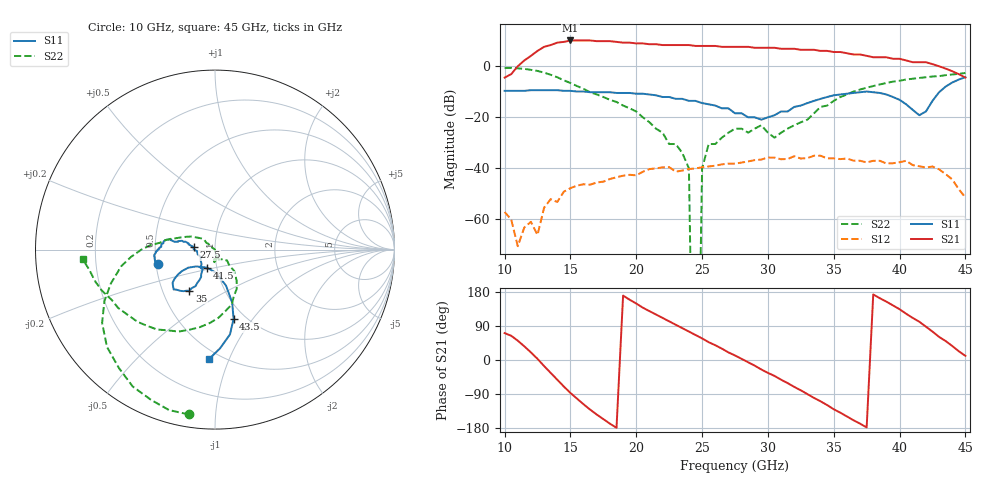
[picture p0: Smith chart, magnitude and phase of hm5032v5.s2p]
!  HMMC-5032
!  S-PARAMETERS at Vdd = 4.5V, Idd = 250mA  LAST UPDATED 03-10-98
#  GHZ  S  MA  R 50
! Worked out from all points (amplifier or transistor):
!   71 points, 10 GHz to 45 GHz, reference 50 ohm
!   highest |S21| = 10.1 dB at 15 GHz (marker M1)
!   |S21| within 3 dB of that: 12.84 GHz to 30.67 GHz (17.83 GHz wide, 81.9 % of centre)
!   unconditionally stable (mu >= 1): start of sweep to end of sweep
!   at 15.5 GHz: K = 25.30, MAG = 11.4 dB, |S12| = -46.7 dB
!   at 27.5 GHz: K = 16.51, MAG = 7.7 dB, |S12| = -38.1 dB
!   at 45 GHz: K = 87.25, MAG = 1.0 dB, |S12| = -51.4 dB
!   S11 on the Smith chart (normalised r, x): 10 GHz: 0.51, -0.09; 27.5 GHz: 0.79, +0.02; 35 GHz: 0.68, -0.34; 41.5 GHz: 0.90, -0.18; 43.5 GHz: 0.88, -0.81; 45 GHz: 0.44, -0.85
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10  0.33 -166.0  0.6 71.0  0.0014 -173.0  0.93 -99.0
11.5  0.33 -167.0  1.3 36.0  0.0007 -143.0  0.89 -121.0
13  0.34 -172.0  2.4 -16.0  0.0017 -134.0  0.75 -147.0
14  0.34 -175.0  2.9 -52.0  0.0022 -168.0  0.61 -162.0
15  0.33 -178.0  3.2 -87.0  0.0041 171.0  0.47 -175.0
16  0.32 -180.0  3.2 -117.0  0.0049 147.0  0.36 176.0
18.5  0.3 177.0  3 -179.0  0.0067 118.0  0.2 160.0
20.5  0.29 171.0  2.8 138.0  0.0086 95.0  0.1 141.0
22  0.25 167.0  2.6 111.0  0.0105 63.0  0.05 139.0
24  0.21 168.0  2.6 75.0  0.0097 45.0  0.01 146.0
24.5  0.21 167.0  2.5 66.0  0.01 41.0  0 -112.0
25  0.19 165.0  2.5 57.0  0.0105 36.0  0.01 -88.0
25.5  0.18 166.0  2.5 47.0  0.0109 30.0  0.03 -72.0
27.5  0.12 173.0  2.4 12.0  0.0124 7.0  0.06 -83.0
30.5  0.11 -133.0  2.3 -42.0  0.0163 -39.0  0.04 -88.0
33.5  0.21 -118.0  2.1 -100.0  0.0177 -90.0  0.12 -48.0
35  0.27 -122.0  1.9 -130.0  0.0157 -115.0  0.21 -55.0
37  0.31 -134.0  1.7 -168.0  0.0141 -152.0  0.35 -81.0
39.5  0.25 -146.0  1.4 144.0  0.0126 160.0  0.5 -114.0
41.5  0.11 -114.0  1.2 101.0  0.011 115.0  0.59 -137.0
43.5  0.4 -75.0  0.9 50.0  0.0077 61.0  0.67 -160.0
45  0.61 -93.0  0.6 11.0  0.0027 59.0  0.74 -176.0
